| TEXAS INSTRUMENTS INCORPORATED
| Standard Linear and Logic Group
| IBIS Model of TWL1200
| SDIO, UART, AND AUDIO VOLTAGE-TRANSLATION TRANSCEIVER
| This file contains package information for the following:
|  WCSP 48-pin (YFF) package as [Component] TWL1200_YFF
| (See IBIS file twl1200_zqc.ibs for BGA-ZQC package information as
|  simulation die data is different)
| This device can be powered at the following Vccs:
|  3.3 volt Vcc
|  2.5 volt Vcc
|  1.8 volt Vcc
|  1.5 volt Vcc
|  1.2 volt Vcc
| This file provides unique models under the [Model Selector] for each Vcc.
| For operation at a specific Vcc, select the appropriate model after each
| [Model Selector] keyword.
[IBIS Ver]   3.2
[Comment char]  |_char
[File Name]   twl1200_yff.ibs
[File Rev]   1.0 | X
[Date]   January 13, 2010
[Source]   Data created from TI-SPICE simulations at TI-SLL.
[Notes]   The following is an IBIS list for the TWL1200.
   Please contact sllibis@ti.com with questions and
   comments concerning SLL IBIS models.
   Note: The IOASDA & IOASDB have a model selector to show the
   different drive levels of the circuit.  The non-_DC model
   demonstrates the full drive circuit used for voltage
   transitions, and the _DC model represents the weaker/low-power
   drive circuit for holding DC levels.
   - FILE REV HISTORY
   - 1.0 Release IBIS file on 1/14/2010
   - Power clamp data deleted was deleted as there is no
   power-clamp diode.
[Disclaimer]
 This model is designed as an aid for customers of Texas Instruments.
 TI and its licensors and suppliers make no warranties, either expressed
 or implied, with respect to this  model, including the warranties of
 merchantability or fitness for a particular purpose.
 The model is provided solely on an "as is" basis. The entire risk as to
 its quality and performance is with the customer.
[Copyright] (C)Copyright 2009 Texas Instruments Incorporated.
   All rights reserved.
| Component TWL1200_YFF 48-PIN WCSP
[Component]   TWL1200_YFF
[Manufacturer]   Texas Instruments, Inc.
[Package]
|   typ   min   max
R_pkg   1.000e-03   1.000e-03   1.000e-03
L_pkg   2.500e-11   2.500e-11   2.500e-11
C_pkg   1.400e-14   1.400e-14   1.400e-14
[Pin]   signal_name   model_name   R_pin   L_pin   C_pin
A1   SDIO_CLK_A AIN   1.000e-03   2.500e-11   1.400e-14
A2   SDIO_CMD_A IOASDA   1.000e-03   2.500e-11   1.400e-14
A3   AUDIO_CLK_A AIO_4MA   1.000e-03   2.500e-11   1.400e-14
A4   AUD_DIR   CONTROLIN   1.000e-03   2.500e-11   1.400e-14
A5   AUDIO_CLK_B BIO_4MA   1.000e-03   2.500e-11   1.400e-14
A6   SDIO_CMD_B IOASDB   1.000e-03   2.500e-11   1.400e-14
A7   SDIO_CLK_B BOUT_8MA   1.000e-03   2.500e-11   1.400e-14
B1   SDIO_DATA3_A IOASDA   1.000e-03   2.500e-11   1.400e-14
B2   SDIO_DATA0_A IOASDA   1.000e-03   2.500e-11   1.400e-14
B3   AUDIO_FSYNC_A AOUT_4MA   1.000e-03   2.500e-11   1.400e-14
B4   OE   CONTROLIN   1.000e-03   2.500e-11   1.400e-14
B5   AUDIO_FSYNC_B BIN   1.000e-03   2.500e-11   1.400e-14
B6   SDIO_DATA0_B IOASDB   1.000e-03   2.500e-11   1.400e-14
B7   SDIO_DATA3_B IOASDB   1.000e-03   2.500e-11   1.400e-14
C1   SDIO_DATA2_A IOASDA   1.000e-03   2.500e-11   1.400e-14
C2   SDIO_DATA1_A IOASDA   1.000e-03   2.500e-11   1.400e-14
C4   VCCA   POWER   1.000e-03   2.500e-11   1.400e-14
C5   VCCB   POWER   1.000e-03   2.500e-11   1.400e-14
C6   SDIO_DATA1_B IOASDB   1.000e-03   2.500e-11   1.400e-14
C7   SDIO_DATA2_B IOASDB   1.000e-03   2.500e-11   1.400e-14
D1   WLAN_EN_A  AIN   1.000e-03   2.500e-11   1.400e-14
D2   WLAN_IRQ_A AOUT_4MA   1.000e-03   2.500e-11   1.400e-14
D3   GND   GND   1.000e-03   2.500e-11   1.400e-14
D4   VCCA   POWER   1.000e-03   2.500e-11   1.400e-14
D5   VCCB   POWER   1.000e-03   2.500e-11   1.400e-14
D6   WLAN_EN_B  BOUT_2MA   1.000e-03   2.500e-11   1.400e-14
D7   WLAN_IRQ_B BIN   1.000e-03   2.500e-11   1.400e-14
E1   CLK_REQ_A  AOUT_8MA   1.000e-03   2.500e-11   1.400e-14
E2   BT_EN_A   AIN   1.000e-03   2.500e-11   1.400e-14
E3   GND   GND   1.000e-03   2.500e-11   1.400e-14
E4   GND   GND   1.000e-03   2.500e-11   1.400e-14
E5   GND   GND   1.000e-03   2.500e-11   1.400e-14
E6   BT_EN_B   BOUT_4MA   1.000e-03   2.500e-11   1.400e-14
E7   CLK_REQ_B  BIN   1.000e-03   2.500e-11   1.400e-14
F1   BT_UART_CTS_A AIN   1.000e-03   2.500e-11   1.400e-14
F2   BT_UART_RTS_A AOUT_4MA   1.000e-03   2.500e-11   1.400e-14
F3   AUDIO_IN_A AIN   1.000e-03   2.500e-11   1.400e-14
F4   SLOW_CLK_B BOUT_2MA   1.000e-03   2.500e-11   1.400e-14
F5   AUDIO_IN_B BOUT_4MA   1.000e-03   2.500e-11   1.400e-14
F6   BT_UART_RTS_B BIN   1.000e-03   2.500e-11   1.400e-14
F7   BT_UART_CTS_B BOUT_4MA   1.000e-03   2.500e-11   1.400e-14
G1   BT_UART_RX_A AIN   1.000e-03   2.500e-11   1.400e-14
G2   BT_UART_TX_A AOUT_8MA   1.000e-03   2.500e-11   1.400e-14
G3   AUD_OUT_A  AOUT_4MA   1.000e-03   2.500e-11   1.400e-14
G4   SLOW_CLK_A AIN   1.000e-03   2.500e-11   1.400e-14
G5   AUD_OUT_B  BIN   1.000e-03   2.500e-11   1.400e-14
G6   BT_UART_TX_B BIN   1.000e-03   2.500e-11   1.400e-14
G7   BT_UART_RX_B BOUT_8MA   1.000e-03   2.500e-11   1.400e-14
| Model BIO_4MA
[Model Selector]   BIO_4MA
BIO_4MA_33   3.3 volt Vcc
BIO_4MA_25   2.5 volt Vcc
BIO_4MA_18   1.8 volt Vcc
BIO_4MA_15A   1.5 volt Vcc
BIO_4MA_12   1.2 volt Vcc
| Model CONTROLIN
[Model Selector]   CONTROLIN
CONTROLIN_33   3.3 volt Vcc
CONTROLIN_25   2.5 volt Vcc
CONTROLIN_18   1.8 volt Vcc
CONTROLIN_15A   1.5 volt Vcc
CONTROLIN_12   1.2 volt Vcc
| Model AIN
[Model Selector]   AIN
AIN_33   3.3 volt Vcc
AIN_25   2.5 volt Vcc
AIN_18   1.8 volt Vcc
AIN_15A   1.5 volt Vcc
AIN_12   1.2 volt Vcc
| Model BIN
[Model Selector]   BIN
BIN_33   3.3 volt Vcc
BIN_25   2.5 volt Vcc
BIN_18   1.8 volt Vcc
BIN_15A   1.5 volt Vcc
BIN_12   1.2 volt Vcc
| Model IOASDB
[Model Selector]   IOASDB
IOASDB_33   3.3 volt Vcc
IOASDB_25   2.5 volt Vcc
IOASDB_18   1.8 volt Vcc
IOASDB_15A   1.5 volt Vcc
IOASDB_12   1.2 volt Vcc
IOASDB_DC_33   3.3 volt Vcc   DC drive only
IOASDB_DC_25   2.5 volt Vcc   DC drive only
IOASDB_DC_18   1.8 volt Vcc   DC drive only
IOASDB_DC_15A   1.5 volt Vcc   DC drive only
IOASDB_DC_12   1.2 volt Vcc   DC drive only
| Model IOASDA
[Model Selector]   IOASDA
IOASDA_33   3.3 volt Vcc
IOASDA_25   2.5 volt Vcc
IOASDA_18   1.8 volt Vcc
IOASDA_15A   1.5 volt Vcc
IOASDA_12   1.2 volt Vcc
IOASDA_DC_33   3.3 volt Vcc   DC drive only
IOASDA_DC_25   2.5 volt Vcc   DC drive only
IOASDA_DC_18   1.8 volt Vcc   DC drive only
IOASDA_DC_15A   1.5 volt Vcc   DC drive only
IOASDA_DC_12   1.2 volt Vcc   DC drive only
| Model BOUT_8MA
[Model Selector]   BOUT_8MA
BOUT_8MA_33   3.3 volt Vcc
BOUT_8MA_25   2.5 volt Vcc
BOUT_8MA_18   1.8 volt Vcc
BOUT_8MA_15A   1.5 volt Vcc
BOUT_8MA_12   1.2 volt Vcc
| Model AIO_4MA
[Model Selector]   AIO_4MA
AIO_4MA_33   3.3 volt Vcc
AIO_4MA_25   2.5 volt Vcc
AIO_4MA_18   1.8 volt Vcc
AIO_4MA_15A   1.5 volt Vcc
AIO_4MA_12   1.2 volt Vcc
| Model AOUT_8MA
[Model Selector]   AOUT_8MA
AOUT_8MA_33   3.3 volt Vcc
AOUT_8MA_25   2.5 volt Vcc
AOUT_8MA_18   1.8 volt Vcc
AOUT_8MA_15A   1.5 volt Vcc
AOUT_8MA_12   1.2 volt Vcc
| Model AOUT_4MA
[Model Selector]   AOUT_4MA
AOUT_4MA_33   3.3 volt Vcc
AOUT_4MA_25   2.5 volt Vcc
AOUT_4MA_18   1.8 volt Vcc
AOUT_4MA_15A   1.5 volt Vcc
AOUT_4MA_12   1.2 volt Vcc
| Model BOUT_4MA
[Model Selector]   BOUT_4MA
BOUT_4MA_33   3.3 volt Vcc
BOUT_4MA_25   2.5 volt Vcc
BOUT_4MA_18   1.8 volt Vcc
BOUT_4MA_15A   1.5 volt Vcc
BOUT_4MA_12   1.2 volt Vcc
| Model BOUT_2MA
[Model Selector]   BOUT_2MA
BOUT_2MA_33   3.3 volt Vcc
BOUT_2MA_25   2.5 volt Vcc
BOUT_2MA_18   1.8 volt Vcc
BOUT_2MA_15A   1.5 volt Vcc
BOUT_2MA_12   1.2 volt Vcc
| Models and submodels in the file (70): BIO_4MA_33 (Input), BIO_4MA_25 (Input), BIO_4MA_18 (Input), BIO_4MA_15A (Input), BIO_4MA_12 (Input), CONTROLIN_33 (Input), CONTROLIN_25 (Input), CONTROLIN_18 (Input), CONTROLIN_15A (Input), CONTROLIN_12 (Input), AIN_33 (Input), AIN_25 (Input), AIN_18 (Input), AIN_15A (Input), AIN_12 (Input), BIN_33 (Input), BIN_25 (Input), BIN_18 (Input), BIN_15A (Input), BIN_12 (Input), IOASDB_33 (I/O), IOASDB_25 (I/O), IOASDB_18 (I/O), IOASDB_15A (I/O), IOASDB_12 (I/O), IOASDA_DC_33 (I/O), IOASDA_DC_25 (I/O), IOASDA_DC_18 (I/O), IOASDA_DC_15A (I/O), IOASDA_DC_12 (I/O), IOASDA_33 (I/O), IOASDA_25 (I/O), IOASDA_18 (I/O), IOASDA_15A (I/O), IOASDA_12 (I/O), IOASDB_DC_33 (I/O), IOASDB_DC_25 (I/O), IOASDB_DC_18 (I/O), IOASDB_DC_15A (I/O), IOASDB_DC_12 (I/O), BOUT_8MA_33 (Output), BOUT_8MA_25 (Output), BOUT_8MA_18 (Output), BOUT_8MA_15A (Output), BOUT_8MA_12 (Output), AIO_4MA_33 (Output), AIO_4MA_25 (Output), AIO_4MA_18 (Output), AIO_4MA_15A (Output), AIO_4MA_12 (Output), AOUT_8MA_33 (Output), AOUT_8MA_25 (Output), AOUT_8MA_18 (Output), AOUT_8MA_15A (Output), AOUT_8MA_12 (Output), AOUT_4MA_33 (Output), AOUT_4MA_25 (Output), AOUT_4MA_18 (Output), AOUT_4MA_15A (Output), AOUT_4MA_12 (Output), BOUT_4MA_33 (Output), BOUT_4MA_25 (Output), BOUT_4MA_18 (Output), BOUT_4MA_15A (Output), BOUT_4MA_12 (Output), BOUT_2MA_33 (Output), BOUT_2MA_25 (Output), BOUT_2MA_18 (Output), BOUT_2MA_15A (Output), BOUT_2MA_12 (Output)
